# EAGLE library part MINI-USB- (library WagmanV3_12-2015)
MINI USB Connector Source: http://www.hirose.co.jp/cataloge_hp/e24000019.pdf
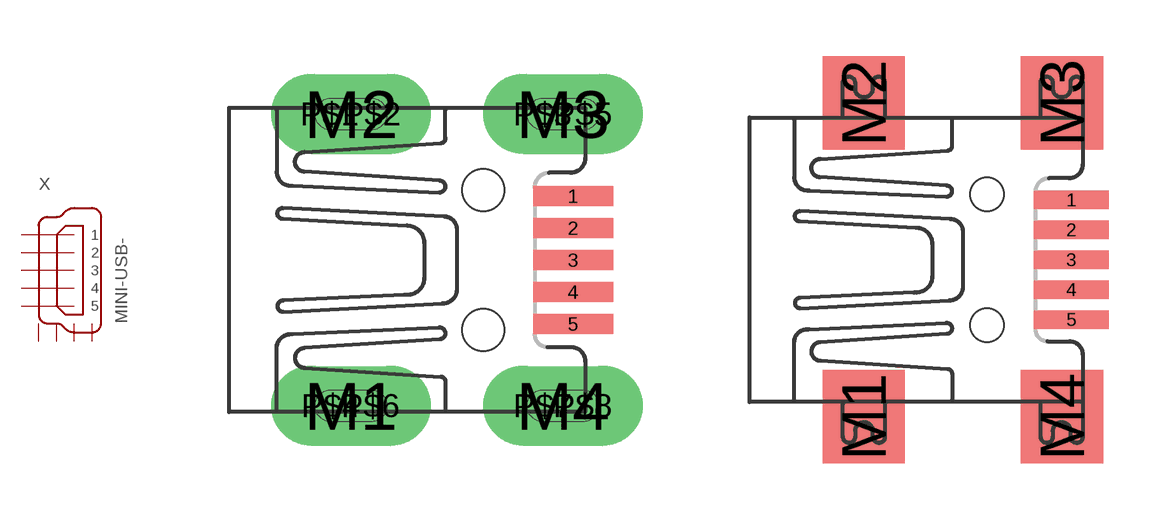
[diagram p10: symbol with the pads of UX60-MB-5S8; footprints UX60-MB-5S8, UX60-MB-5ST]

Designator prefix X

## MINI-USB-UX60-MB-5S8 (OC_FARNELL: unknown; OC_NEWARK: unknown)  [UX60-MB-5S8]
1  1  in
2  2  in
3  3  in
4  4  in
5  5  in
M1  M1  in
M2  M2  in
M3  M3  in
M4  M4  in

## MINI-USB-UX60-MB-5ST (OC_FARNELL: unknown; OC_NEWARK: unknown)  [UX60-MB-5ST]
Pads as for UX60-MB-5S8

## MINI-USB-UX60A-MB-5ST (OC_FARNELL: unknown; OC_NEWARK: unknown)  [UX60A-MB-5ST]
Pads as for UX60-MB-5S8

## Footprint UX60-MB-5S8 (pad centres in mm)
MINI USB Connector HI-SPEED Certified Metal Shield Dip Type With Positioning Post Source: http://www.hirose.co.jp/cataloge_hp/e24000019.pdf
smd 2 x 0.5: 1 8.65,1.6; 2 8.65,0.8; 3 8.65,0; 4 8.65,-0.8; 5 8.65,-1.6
drill 0.8 pad 2 long: M1 3.1,-3.65; M2 3.1,3.65; M3 8.4,3.65; M4 8.4,-3.65
drill 0.8: P$1 2.57,3.65; P$2 3.62,3.65; P$3 7.895,3.65; P$4 2.595,-3.65; P$5 8.895,3.65; P$6 3.595,-3.65; P$7 7.895,-3.65; P$8 8.895,-3.65
hole 1.05 at 6.4,-1.75
hole 1.05 at 6.4,1.75

## Footprint UX60-MB-5ST (pad centres in mm)
MINI USB Connector HI-SPEED Certified Metal Shield SMT Type With Positioning Post Source: http://www.hirose.co.jp/cataloge_hp/e24000019.pdf
smd 2 x 0.5: 1 2.25,1.6; 2 2.25,0.8; 3 2.25,0; 4 2.25,-0.8; 5 2.25,-1.6
smd 2.2 x 2.5: M1 -3.3,-4.2; M2 -3.3,4.2; M3 2,4.2; M4 2,-4.2
hole 0.9 at 0,-1.75
hole 0.9 at 0,1.75

## Footprint UX60A-MB-5ST (pad centres in mm)
MINI USB Connector HI-SPEED Certified Metal Shield SMT Type Without Positioning Post Source: http://www.hirose.co.jp/cataloge_hp/e24000019.pdf
smd 2 x 0.5: 1 2.25,1.6; 2 2.25,0.8; 3 2.25,0; 4 2.25,-0.8; 5 2.25,-1.6
smd 2.2 x 2.5: M1 -3.3,-4.2; M2 -3.3,4.2; M3 2,4.2; M4 2,-4.2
